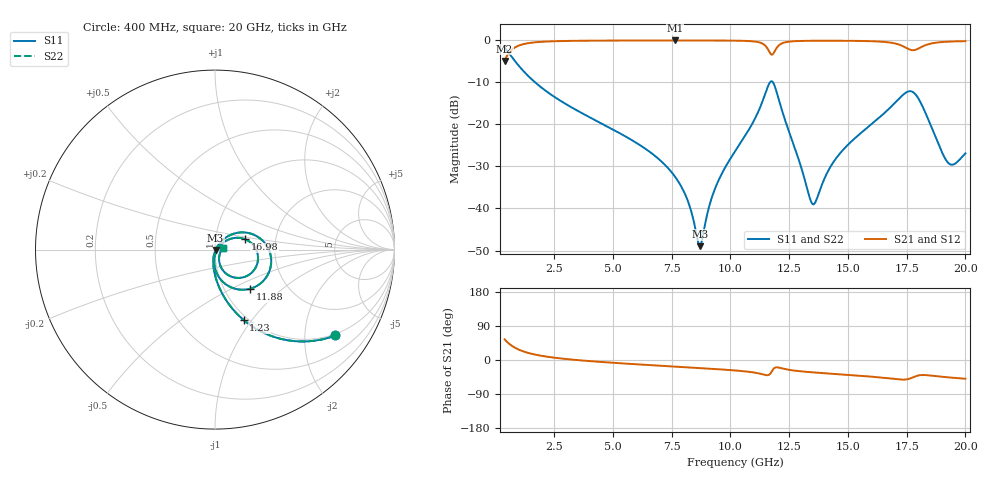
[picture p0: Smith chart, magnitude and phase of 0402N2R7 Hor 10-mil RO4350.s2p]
# GHz S MA R 50
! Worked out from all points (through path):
!   1960 points, 400 MHz to 20 GHz, reference 50 ohm
!   highest |S21| = -0.03 dB at 7.654 GHz (marker M1); lowest = -4.9 dB at 400 MHz (marker M2)
!   group delay of S21, straight-line fit = 9.92 ps
!   lowest |S11| = -49.0 dB at 8.704 GHz (marker M3), VSWR 1.01, Z = 50.3 - j0.145 ohm
!   |S11| at or under -10 dB: 1.699 GHz to 11.69 GHz (9.988 GHz wide, 149 % of centre); 11.82 GHz to end of sweep
!   |S22| runs from -49.0 to -1.7 dB; largest |S21 - S12| = 0
!   S11 on the Smith chart (normalised r, x): 400 MHz: 0.95, -2.83; 1.23 GHz: 0.95, -0.91; 11.88 GHz: 1.31, -0.63; 16.98 GHz: 1.39, +0.17; 20 GHz: 1.09, +0.02
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0.4  0.8236 -35.5  0.5668 54.5  0.5668 54.5  0.8236 -35.5
0.8002042  0.5857 -56.1  0.8099 33.9  0.8099 33.9  0.5857 -56.1
1.230424  0.4225 -67.9  0.9054 22.0  0.9054 22.0  0.4225 -67.9
3.671669  0.1369 -90.5  0.9887 -1.2  0.9887 -1.2  0.1369 -90.5
6.943338  0.03898 -101.0  0.9964 -14.8  0.9964 -14.8  0.03898 -101.0
7.653701  0.02379 -100.5  0.9965 -17.4  0.9965 -17.4  0.02379 -100.5
8.193977  0.01229 -94.5  0.9964 -19.4  0.9964 -19.4  0.01229 -94.5
8.704237  0.003562 -23.9  0.9961 -21.3  0.9961 -21.3  0.003562 -23.9
9.324553  0.01649 51.0  0.9951 -23.7  0.9951 -23.7  0.01649 51.0
10.205  0.04797 53.5  0.991 -27.6  0.991 -27.6  0.04797 53.5
11.43563  0.2111 25.7  0.8902 -38.8  0.8902 -38.8  0.2111 25.7
11.69576  0.3187 -10.7  0.7025 -36.3  0.7025 -36.3  0.3187 -10.7
11.87586  0.2922 -48.4  0.7309 -21.1  0.7309 -21.1  0.2922 -48.4
12.26605  0.1277 -86.4  0.9355 -23.2  0.9355 -23.2  0.1277 -86.4
13.46667  0.0116 -41.0  0.988 -32.4  0.988 -32.4  0.0116 -41.0
14.64727  0.04461 39.6  0.9887 -37.7  0.9887 -37.7  0.04461 39.6
16.73834  0.1524 25.3  0.9457 -48.4  0.9457 -48.4  0.1524 25.3
16.97846  0.1777 18.9  0.9216 -50.1  0.9216 -50.1  0.1777 18.9
17.78887  0.2403 -33.2  0.7629 -45.2  0.7629 -45.2  0.2403 -33.2
18.36917  0.124 -69.1  0.8889 -40.1  0.8889 -40.1  0.124 -69.1
19.23961  0.0356 -41.4  0.9637 -45.6  0.9637 -45.6  0.0356 -41.4
20  0.04526 13.0  0.9775 -49.5  0.9775 -49.5  0.04526 13.0
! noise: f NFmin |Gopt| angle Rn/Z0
0.4  0.001254  0.7905  3.373  0.001232
2.571  0.005048  0.6778  7.278  0.003015
4.752  0.00809  0.6382  12.26  0.004172
6.933  0.01112  0.6221  17.27  0.005377
9.104  0.01574  0.6471  22.18  0.008157
11.29  0.0629  0.8766  27.33  0.104
13.47  0.03172  0.7337  32.51  0.02195
15.64  0.03769  0.7422  37.27  0.0264
17.82  0.1826  0.9337  42.37  0.5332
20  0.05117  0.7621  47.06  0.03681
